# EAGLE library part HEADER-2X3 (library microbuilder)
PIN HEADER
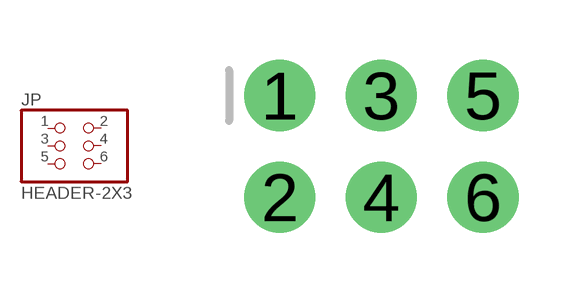
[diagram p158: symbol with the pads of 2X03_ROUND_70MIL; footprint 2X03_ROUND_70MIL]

Designator prefix JP

## HEADER-2X3  [2X03_ROUND_70MIL]
1  1  pas
2  2  pas
3  3  pas
4  4  pas
5  5  pas
6  6  pas

## Footprint 2X03_ROUND_70MIL (pad centres in mm)
drill 1 pad 1.778: 1 -2.54,1.27; 2 -2.54,-1.27; 3 0,1.27; 4 0,-1.27; 5 2.54,1.27; 6 2.54,-1.27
